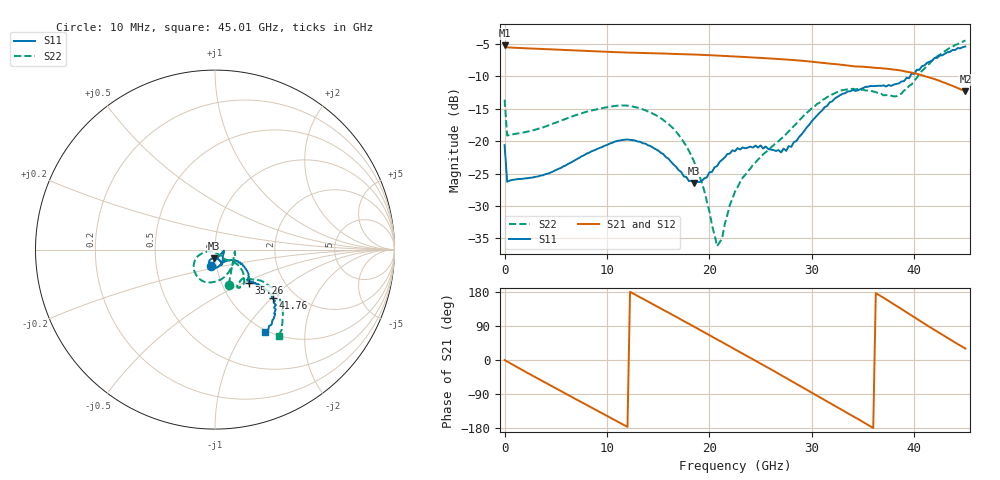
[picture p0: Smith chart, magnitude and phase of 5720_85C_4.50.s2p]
! Device:  ADRF5720
! Description: 0.5dB LSB GaAs MMIC 6-bit Digital Attenuator
! Frequency:  0.000009 -  40 GHz
! Ports:
!	RF1	= Port 1
!	RF2	= Port 2
! Vdd:  3.3 Volt
! Vss:  -3.3 Volt
! Control:  0/3.3 Volt
! State:  4.50 dB attenuation
! Data:  The device was measured using G-S-G Probes on a matrix board.
!  Data was collected using an calibrated 4 port network analyzer.
!  The reference plane for this measurement is at the launchers.
! Note:  Analog Devices supplies this data as a sample of measured data
!  for this product.  Your particular data for this product may vary.
!  Data was taken at 85 degrees C.
!  Analog Devices reserves the right to change this data at anytime.
# GHZ S DB R 45.0
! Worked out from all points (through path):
!   181 points, 10 MHz to 45.01 GHz, reference 45 ohm
!   highest |S21| = -5.18 dB at 10 MHz (marker M1); lowest = -12.3 dB at 45.01 GHz (marker M2)
!   group delay of S21, straight-line fit = 42.2 ps
!   lowest |S11| = -26.4 dB at 18.51 GHz (marker M3), VSWR 1.10, Z = 44.5 - j4.24 ohm
!   |S11| at or under -10 dB: start of sweep to 39.6 GHz
!   |S22| runs from -36.2 to -4.4 dB; largest |S21 - S12| = 0.0028
!   S11 on the Smith chart (normalised r, x): 10 MHz: 0.94, -0.17; 35.26 GHz: 1.34, -0.53; 41.76 GHz: 1.54, -1.01; 45.01 GHz: 0.98, -1.26
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0.01  -20.61 -105.6  -5.18 -0.1  -5.17 -0.1  -13.59 -68.5
0.26  -26.26 -9.3  -5.50 -4.0  -5.49 -4.0  -19.12 -5.5
2.26  -25.70 -19.7  -5.66 -34.2  -5.64 -34.1  -18.51 -22.8
4.26  -25.00 -38.5  -5.79 -63.7  -5.77 -63.7  -17.58 -44.7
7.76  -22.18 -58.3  -6.04 -114.9  -6.02 -114.8  -15.56 -75.8
11.51  -19.80 -88.2  -6.28 -169.3  -6.27 -169.2  -14.47 -108.7
15.26  -21.78 -114.2  -6.45 136.0  -6.43 136.2  -16.45 -142.2
17.26  -24.75 -112.8  -6.55 106.6  -6.53 106.7  -19.53 -158.2
18.51  -26.43 -94.4  -6.61 88.0  -6.60 88.2  -23.17 -165.0
19.51  -25.74 -77.8  -6.68 73.1  -6.66 73.2  -27.66 -165.3
20.76  -23.83 -66.8  -6.77 54.4  -6.75 54.6  -36.20 -120.6
21.26  -22.85 -66.0  -6.81 46.9  -6.79 47.1  -34.96 -78.7
22.76  -21.06 -65.3  -6.94 24.4  -6.92 24.6  -27.09 -48.0
25.01  -20.65 -67.0  -7.14 -9.4  -7.12 -9.2  -22.46 -45.0
27.51  -21.49 -47.2  -7.38 -47.5  -7.37 -47.2  -18.89 -33.4
30.26  -16.48 -28.8  -7.77 -90.0  -7.75 -89.7  -14.68 -36.8
32.51  -13.15 -34.4  -8.12 -124.8  -8.10 -124.5  -12.39 -47.2
35.26  -11.61 -44.4  -8.53 -167.5  -8.51 -167.2  -12.16 -59.0
37.76  -11.46 -41.7  -8.89 151.7  -8.87 152.0  -12.97 -50.2
39.76  -9.54 -38.8  -9.40 117.4  -9.37 117.8  -11.23 -37.6
41.76  -7.53 -40.2  -10.30 83.3  -10.28 83.7  -7.55 -34.7
45.01  -5.38 -58.5  -12.29 30.2  -12.26 30.6  -4.44 -53.3
